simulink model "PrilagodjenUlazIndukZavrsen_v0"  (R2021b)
settings: Solver=VariableStepAuto  StartTime=0.0  StopTime=200e-09  MaxStep=1e-9  RelTol=1e-3
libraries: fl_lib x9, nesl_utility x5, simulink x1, ee_lib x1

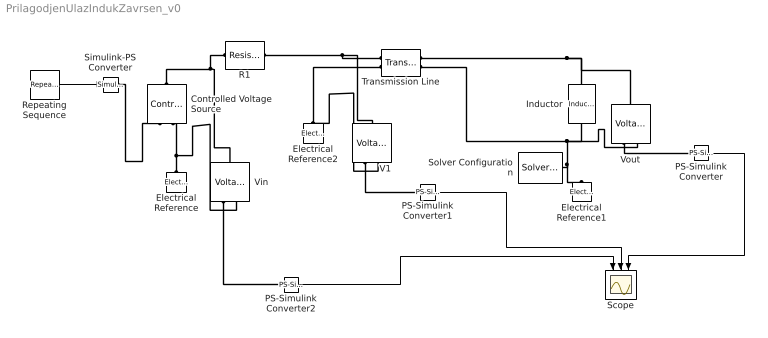
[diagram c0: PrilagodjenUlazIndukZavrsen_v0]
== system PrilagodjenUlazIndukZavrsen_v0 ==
  Controlled Voltage Source : fl_lib/Electrical/Electrical Sources/Controlled Voltage Source
  Electrical Reference : fl_lib/Electrical/Electrical Elements/Electrical Reference
  Electrical Reference1 : fl_lib/Electrical/Electrical Elements/Electrical Reference
  Electrical Reference2 : fl_lib/Electrical/Electrical Elements/Electrical Reference
  Inductor : fl_lib/Electrical/Electrical Elements/Inductor  l=200 nH  r=0 Ohm  g=1e-9 1/Ohm  i_specify=off  i_priority=None  i=0 A  i_nominal_specify=off  i_nominal_unit=A  i_nominal_value=1  v_specify=off  v_priority=None  v=0 V  v_nominal_specify=off  v_nominal_unit=V  v_nominal_value=1  i_L_specify=off  i_L_priority=High  i_L=0 A  i_L_nominal_specify=off  i_L_nominal_unit=A  i_L_nominal_value=1
  PS-Simulink Converter : nesl_utility/PS-Simulink Converter  PhysicalDomain=network_engine_domain  SubClassName=ps_output  LeftPortType=input  RightPortType=output  PseudoPeriodic=off  Frequencies=[]  Unit=inherit  AffineConversion=off
  PS-Simulink Converter1 : nesl_utility/PS-Simulink Converter  PhysicalDomain=network_engine_domain  SubClassName=ps_output  LeftPortType=input  RightPortType=output  PseudoPeriodic=off  Frequencies=[]  Unit=inherit  AffineConversion=off
  PS-Simulink Converter2 : nesl_utility/PS-Simulink Converter  PhysicalDomain=network_engine_domain  SubClassName=ps_output  LeftPortType=input  RightPortType=output  PseudoPeriodic=off  Frequencies=[]  Unit=inherit  AffineConversion=off
  R1 : fl_lib/Electrical/Electrical Elements/Resistor  R=50 Ohm  i_specify=off  i_priority=None  i=0 A  i_nominal_specify=off  i_nominal_unit=A  i_nominal_value=1  v_specify=off  v_priority=None  v=0 V  v_nominal_specify=off  v_nominal_unit=V  v_nominal_value=1
  Repeating Sequence : simulink/Sources/Repeating Sequence  rep_seq_t=[0 1 20 21 300]*1e-9  rep_seq_y=[0 1 1 0 0]
  Scope : Scope  NumInputPorts=3
  Simulink-PS Converter : nesl_utility/Simulink-PS Converter  PhysicalDomain=network_engine_domain  SubClassName=ps_input  LeftPortType=input  RightPortType=output  PseudoPeriodic=off  Frequencies=[]  NoiseDistribution=none  NoiseParameters=[]  Unit=1  AffineConversion=off  FilteringAndDerivatives=provide  SimscapeFilterOrder=1  InputFilterTimeConstant=0.001  UdotUserProvided=0
  Solver Configuration : nesl_utility/Solver Configuration  PhysicalDomain=network_engine_domain  SubClassName=solver  LeftPortType=input  RightPortType=generic  Tones=[]  Harmonics=[]  SimulateNoise=off  Profile=off  UseLocalSampling=off  EnableSwitchedLinearOptims=on  FrequencyDomain=off  UseCCode=off  RelTol=0.001  AbsTol=1e-06  MinStep=1e-09  ToWorkspace=off  RevertToSquareIcSolve=off  NumHomotopyIterations=100  PhasorMode=off  PhasorModeNumHarmonics=1  DoDC=off  ResidualTolerance=1e-09  UseLocalSolver=off  LocalSolverChoice=NE_BACKWARD_EULER_ADVANCER  LocalSolverSampleTime=0.001  DoFixedCost=off  MaxNonlinIter=3  MaxModeIter=2  ComputeImpulses=off  ImpulseIterations=2  LinearAlgebra=auto  EquationFormulation=NE_TIME_EF  DelaysMemoryBudget=1024  AutomaticFiltering=on  FilteringTimeConstant=0.001  PartitionStorageMethod=AS_NEEDED  PartitionMemoryBudget=1024  PartitionMethod=ROBUST
  Transmission Line : ee_lib/Passive/Lines/Transmission Line  model_type=1  TD=60 ns  LC_param=1  Z0_delay_based=50 Ohm  Z0=50 Ohm  freq=60 Hz  Ll=220 uH/m  L=220 uH/m  C=90 pF/m  R=0.3 Ohm/m  G=5e-6 S/m  LEN=1 m  N=1
  V1 : fl_lib/Electrical/Electrical Sensors/Voltage Sensor
  Vin : fl_lib/Electrical/Electrical Sensors/Voltage Sensor
  Vout : fl_lib/Electrical/Electrical Sensors/Voltage Sensor
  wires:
  Repeating Sequence/1 -> Simulink-PS Converter/1
  PS-Simulink Converter2/1 -> Scope/1
  PS-Simulink Converter1/1 -> Scope/2
  PS-Simulink Converter/1 -> Scope/3
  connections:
  Electrical Reference2/LConn1 -- V1/RConn2 -- Transmission Line/LConn2
  Transmission Line/RConn2 -- Inductor/RConn1 -- Vout/RConn2 -- Solver Configuration/RConn1 -- Electrical Reference1/LConn1
  Electrical Reference/LConn1 -- Vin/RConn2 -- Controlled Voltage Source/RConn2
  Controlled Voltage Source/LConn1 -- Vin/LConn1 -- R1/LConn1
  R1/RConn1 -- V1/LConn1 -- Transmission Line/LConn1
  Transmission Line/RConn1 -- Inductor/LConn1 -- Vout/LConn1
  Simulink-PS Converter/RConn1 -- Controlled Voltage Source/RConn1
  Vout/RConn1 -- PS-Simulink Converter/LConn1
  V1/RConn1 -- PS-Simulink Converter1/LConn1
  Vin/RConn1 -- PS-Simulink Converter2/LConn1
